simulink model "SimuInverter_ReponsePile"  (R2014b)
settings: Solver=ode45  SolverMode=SingleTasking  StartTime=0.0  StopTime=1  MaxStep=Ts/10  RelTol=1e-8
undefined symbols (not defined in the file): Am, Bm, C, denKfilter, Kz, L, numK, R, Ts
libraries: simulink x3

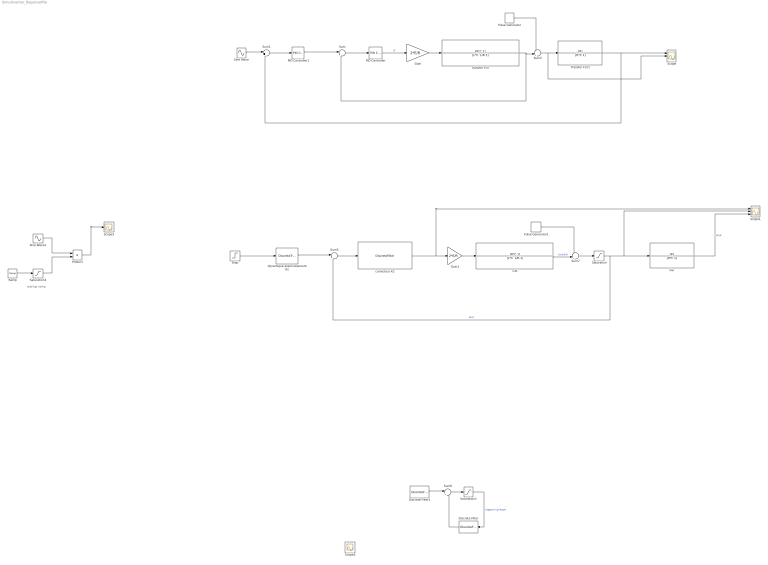
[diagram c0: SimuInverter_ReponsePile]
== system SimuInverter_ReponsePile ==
  note: startup ramp
  Discrete Filter : DiscreteFilter  Commented=on  Numerator=denKfilter  Denominator=1  SampleTime=Ts
  Discrete Filter1 : DiscreteFilter  Commented=on  Numerator=numK  Denominator=1  SampleTime=Ts
  Gain : Gain  Commented=on  Gain=2*E/R
  Gain1 : Gain  Gain=2*E/R
  Gid : TransferFcn  Numerator=[R*C 1]  Denominator="[L*C  L/R 1]"
  Gvi : TransferFcn  Numerator=[R]  Denominator=[R*C 1]
  PID Controller : simulink/Continuous/PID Controller  Commented=on  Controller=PI  Form=Ideal  TimeDomain=Continuous-time  SampleTime=-1  IntegratorMethod=Forward Euler  FilterMethod=Forward Euler  ControllerParametersSource=internal  P=0.0397660737840984  I=621539.214990914  D=0  UseFilter=on  N=100  InitialConditionSource=internal  InitialConditionForIntegrator=0  InitialConditionForFilter=0  DifferentiatorICPrevScaledInput=0  ExternalReset=none  TrackingMode=off  Kt=1  LimitOutput=off  UpperSaturationLimit=inf  LowerSaturationLimit=-inf  LinearizeAsGain=on  AntiWindupMode=none  Kb=1  POutMin=[]  POutMax=[]  IOutMin=[]  IOutMax=[]  DOutMin=[]  DOutMax=[]  NOutMin=[]  NOutMax=[]  SumOutMin=[]  SumOutMax=[]  SaturationOutMin=[]  SaturationOutMax=[]  PParamMin=[]  PParamMax=[]  IParamMin=[]  IParamMax=[]  DParamMin=[]  DParamMax=[]  NParamMin=[]  NParamMax=[]  KbParamMin=[]  KbParamMax=[]  KtParamMin=[]  KtParamMax=[]  KbOutMin=[]  KbOutMax=[]  KtOutMin=[]  KtOutMax=[]  IntegratorOutMin=[]  IntegratorOutMax=[]  FilterOutMin=[]  FilterOutMax=[]  SumI1OutMin=[]  SumI1OutMax=[]  SumI2OutMin=[]  SumI2OutMax=[]  SumI3OutMin=[]  SumI3OutMax=[]  SumDOutMin=[]  SumDOutMax=[]  DifferentiatorOutMin=[]  DifferentiatorOutMax=[]  IntegratorContinuousStateAttributes=''  IntegratorStateMustResolveToSignalObject=off  IntegratorRTWStateStorageClass=Auto  FilterContinuousStateAttributes=''  FilterStateMustResolveToSignalObject=off  FilterRTWStateStorageClass=Auto
  PID Controller1 : simulink/Continuous/PID Controller  Commented=on  Controller=PI  Form=Ideal  TimeDomain=Continuous-time  SampleTime=-1  IntegratorMethod=Forward Euler  FilterMethod=Forward Euler  ControllerParametersSource=internal  P=0.153193542705994  I=2920.70140213559  D=0  UseFilter=on  N=100  InitialConditionSource=internal  InitialConditionForIntegrator=0  InitialConditionForFilter=0  DifferentiatorICPrevScaledInput=0  ExternalReset=none  TrackingMode=off  Kt=1  LimitOutput=off  UpperSaturationLimit=inf  LowerSaturationLimit=-inf  LinearizeAsGain=on  AntiWindupMode=none  Kb=1  POutMin=[]  POutMax=[]  IOutMin=[]  IOutMax=[]  DOutMin=[]  DOutMax=[]  NOutMin=[]  NOutMax=[]  SumOutMin=[]  SumOutMax=[]  SaturationOutMin=[]  SaturationOutMax=[]  PParamMin=[]  PParamMax=[]  IParamMin=[]  IParamMax=[]  DParamMin=[]  DParamMax=[]  NParamMin=[]  NParamMax=[]  KbParamMin=[]  KbParamMax=[]  KtParamMin=[]  KtParamMax=[]  KbOutMin=[]  KbOutMax=[]  KtOutMin=[]  KtOutMax=[]  IntegratorOutMin=[]  IntegratorOutMax=[]  FilterOutMin=[]  FilterOutMax=[]  SumI1OutMin=[]  SumI1OutMax=[]  SumI2OutMin=[]  SumI2OutMax=[]  SumI3OutMin=[]  SumI3OutMax=[]  SumDOutMin=[]  SumDOutMax=[]  DifferentiatorOutMin=[]  DifferentiatorOutMax=[]  IntegratorContinuousStateAttributes=''  IntegratorStateMustResolveToSignalObject=off  IntegratorRTWStateStorageClass=Auto  FilterContinuousStateAttributes=''  FilterStateMustResolveToSignalObject=off  FilterRTWStateStorageClass=Auto
  Product : Product
  Pulse Generator : DiscretePulseGenerator  Commented=on  PulseType=Time based  Amplitude=2  Period=0.1  PhaseDelay=0.035
  Pulse Generator1 : DiscretePulseGenerator  Commented=on  PulseType=Time based  Period=10  PhaseDelay=0.2
  Ramp : simulink/Sources/Ramp  slope=1/0.1  start=0  X0=0
  Saturation : Saturate  Commented=through  UpperLimit=10  LowerLimit=-10
  Saturation1 : Saturate  Commented=on
  Saturation3 : Saturate  UpperLimit=1  LowerLimit=0
  Scope : Scope  NumInputPorts=3
  Scope1 : Scope  NumInputPorts=3
  Scope2 : Scope
  Scope3 : Scope
  Sine Wave : Sin  Commented=on  Amplitude=230*sqrt(2)*0.95  Frequency=2*pi*50  SampleTime=0
  Sine Wave1 : Sin  Amplitude=230*sqrt(2)  Frequency=2*pi*50  SampleTime=0
  Step : Step  Time=0.1  After=100  SampleTime=Ts
  Sum : Sum  Commented=on  Inputs=|+-
  Sum1 : Sum  Commented=on  Inputs=|+-
  Sum2 : Sum  Commented=on  Inputs=++|
  Sum3 : Sum  Inputs=|+-
  Sum6 : Sum  Commented=on  Inputs=|+-
  Sum7 : Sum  Inputs=++|
  Transfer Fcn : TransferFcn  Commented=on  Numerator=[R*C 1]  Denominator="[L*C  L/R 1]"
  Transfer Fcn1 : TransferFcn  Commented=on  Numerator=[R]  Denominator=[R*C 1]
  correcteur Kz : DiscreteFilter  Numerator=Kz  Denominator=1  SampleTime=Ts
  dynamique asservissement Gz : DiscreteTransferFcn  Numerator=Bm  Denominator=Am  SampleTime=Ts
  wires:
  Transfer Fcn/1 -> Sum2/2, Sum/2
  Gain/1 -> Transfer Fcn/1
  Transfer Fcn1/1 -> Sum1/2, Scope/1
  Sum1/1 -> PID Controller1/1
  Sine Wave/1 -> Sum1/1
  Pulse Generator/1 -> Sum2/1
  Sum2/1 -> Scope/2, Transfer Fcn1/1
  PID Controller1/1 -> Sum/1
  PID Controller/1 -> Gain/1  "d'"
  Sum/1 -> PID Controller/1
  Gain1/1 -> Gid/1
  Gid/1 -> Sum7/2  "courant"
  Pulse Generator1/1 -> Sum7/1
  Product/1 -> Scope3/1
  Sum7/1 -> Saturation/1
  Saturation/1 -> Scope1/2, Gvi/1, Sum3/2  "Iout"
  Sine Wave1/1 -> Product/1
  Ramp/1 -> Saturation3/1
  Saturation3/1 -> Product/2
  Gvi/1 -> Scope1/3  "Vout"
  dynamique asservissement Gz/1 -> Sum3/1
  Saturation1/1 -> Discrete Filter/1  "rapport cyclique"
  Discrete Filter1/1 -> Sum6/1
  Sum6/1 -> Saturation1/1
  Discrete Filter/1 -> Sum6/2
  Step/1 -> dynamique asservissement Gz/1
  correcteur Kz/1 -> Scope1/1, Gain1/1
  Sum3/1 -> correcteur Kz/1
